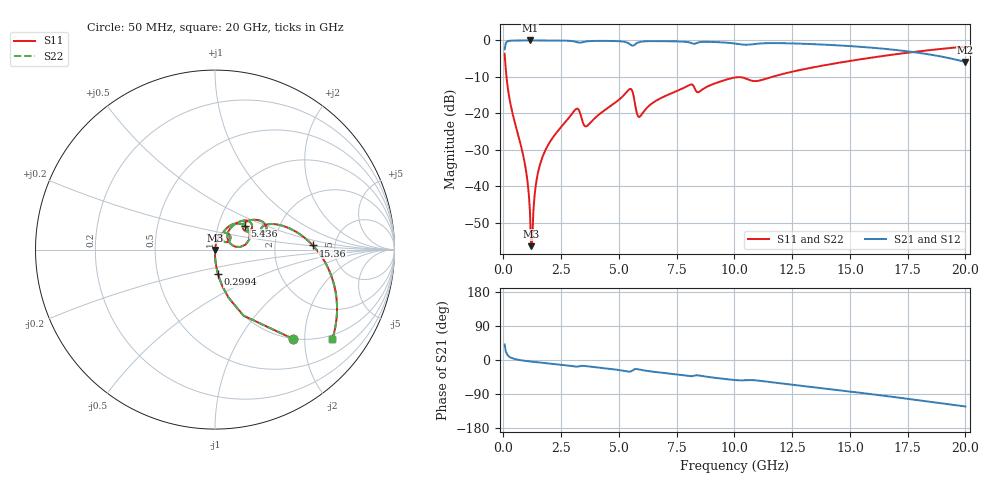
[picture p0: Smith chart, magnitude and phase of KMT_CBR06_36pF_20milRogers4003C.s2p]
! Data measured by Modelithics Inc. support@modelithics.com 813-866-6335
! KEMET CBR0603 36pF, Pad Width= 0.851mm, Pad Length= 0.64mm, Pad Gap= 0.62mm, 20mil Rogers 4003C substrate Data, January 2022
# hz S ma R 50
! 2 Port Network Data from SP1.SP block
! freq  magS11  angS11  magS21  angS21  magS12  angS12  magS22  angS22
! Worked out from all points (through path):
!   401 points, 50 MHz to 20 GHz, reference 50 ohm
!   highest |S21| = -0.01 dB at 1.147 GHz (marker M1); lowest = -5.9 dB at 20 GHz (marker M2)
!   group delay of S21, straight-line fit = 17 ps
!   lowest |S11| = -56.5 dB at 1.197 GHz (marker M3), VSWR 1.00, Z = 50.1 - j0.14 ohm
!   |S11| at or under -10 dB: 132.1 MHz to 11.64 GHz (11.5 GHz wide, 196 % of centre)
!   |S22| runs from -56.5 to -1.7 dB; largest |S21 - S12| = 0
!   S11 on the Smith chart (normalised r, x): 50 MHz: 1.00, -1.75; 299.4 MHz: 1.00, -0.28; 5.436 GHz: 1.33, +0.37; 15.36 GHz: 3.38, +0.23; 20 GHz: 0.88, -2.71
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5e7  0.6595 -48.9  0.7512 41.1  0.7512 41.1  0.6595 -48.9
2.99375e8  0.1368 -83.0  0.9902 6.8  0.9902 6.8  0.1368 -83.0
9.4775e8  0.0186 -90.5  0.9992 -2.3  0.9992 -2.3  0.0186 -90.5
1.0475e9  0.01119 -90.0  0.9993 -3.1  0.9993 -3.1  0.01119 -90.0
1.14725e9  0.004527 -85.7  0.9993 -3.8  0.9993 -3.8  0.004527 -85.7
1.197125e9  0.001504 -68.4  0.9993 -4.2  0.9993 -4.2  0.001504 -68.4
1.296875e9  0.004614 76.5  0.9993 -4.9  0.9993 -4.9  0.004614 76.5
1.396625e9  0.01014 80.3  0.9992 -5.5  0.9992 -5.5  0.01014 80.3
1.496375e9  0.01542 80.9  0.9991 -6.2  0.9991 -6.2  0.01542 80.9
1.8455e9  0.03261 79.9  0.9984 -8.4  0.9984 -8.4  0.03261 79.9
3.092375e9  0.1107 58.2  0.9661 -17.1  0.9661 -17.1  0.1107 58.2
3.391625e9  0.08369 30.9  0.9404 -15.5  0.9404 -15.5  0.08369 30.9
3.641e9  0.06782 53.0  0.9741 -16.6  0.9741 -16.6  0.06782 53.0
5.4365e9  0.2124 39.2  0.9067 -30.7  0.9067 -30.7  0.2124 39.2
5.885375e9  0.08923 32.7  0.9494 -25.1  0.9494 -25.1  0.08923 32.7
6.73325e9  0.1567 53.7  0.9778 -32.8  0.9778 -32.8  0.1567 53.7
1.0025e10  0.3103 28.8  0.9066 -52.9  0.9066 -52.9  0.3103 28.8
1.10225e10  0.279 23.7  0.9036 -54.3  0.9036 -54.3  0.279 23.7
1.336662e10  0.4247 16.7  0.8904 -71.4  0.8904 -71.4  0.4247 16.7
1.536162e10  0.5454 2.5  0.8217 -85.9  0.8217 -85.9  0.5454 2.5
1.670825e10  0.6291 -8.1  0.7559 -96.1  0.7559 -96.1  0.6291 -8.1
2e10  0.8218 -37.3  0.5062 -122.7  0.5062 -122.7  0.8218 -37.3
